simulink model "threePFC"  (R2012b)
settings: Solver=ode15s  StartTime=0.0  StopTime=0.1  MaxStep=1e-6  RelTol=1e-4
libraries: powerlib x29, simulink x10

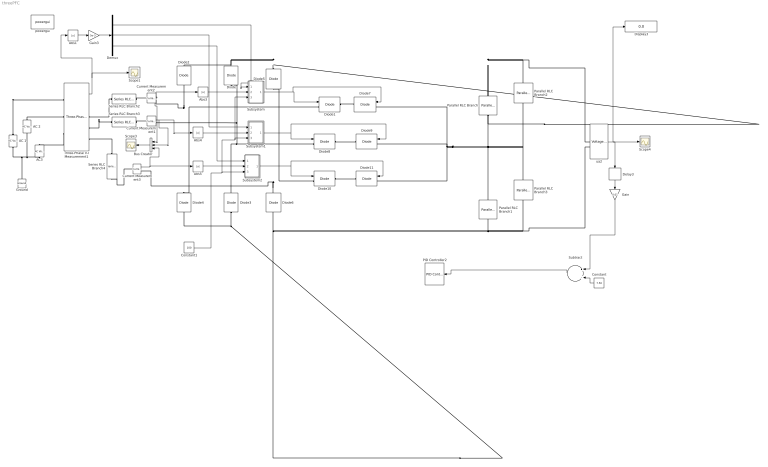
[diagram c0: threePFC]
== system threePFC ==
  AC 1 : powerlib/Electrical Sources/AC Voltage Source  Amplitude=200  Phase=0  Frequency=50  SampleTime=0  Measurements=Voltage
  AC 2 : powerlib/Electrical Sources/AC Voltage Source  Amplitude=200  Phase=120  Frequency=50  SampleTime=0  Measurements=None
  AC3 : powerlib/Electrical Sources/AC Voltage Source  Amplitude=200  Phase=240  Frequency=50  SampleTime=0  Measurements=None
  Abs{1,3..5} (4 alike) : Abs
  Bus Creator : BusCreator  Inputs=3
  Constant : Constant  Value=7.50
  Constant1 : Constant  Value=100
  Current Measurement1 : powerlib/Measurements/Current Measurement  PhasorSimulation=off  OutputType=Complex  PSBequivalent=0
  Current Measurement2 : powerlib/Measurements/Current Measurement  PhasorSimulation=off  OutputType=Complex  PSBequivalent=0
  Current Measurement3 : powerlib/Measurements/Current Measurement  PhasorSimulation=off  OutputType=Complex  PSBequivalent=0
  Delay3 : Delay  DelayLength=1  InitialCondition=0  SampleTime=1e-6
  Demux : Demux  Outputs=3
  Diode{,2..6} (6 alike) : powerlib/Power Electronics/Diode  Ron=0.001  Lon=0  Vf=0.8  IC=0  UseSnubber=off  Rs=500  Cs=250e-9  Measurements=off
  Diode{1,7..11} (6 alike) : powerlib/Power Electronics/IGBT//Diode  Ron=1e-3  Rs=1e5  Cs=inf  Measurements=off
  Display3 : Display
  Gain : Gain  Gain=0.01
  Gain3 : Gain  Gain=5e-3
  Ground : powerlib/Elements/Ground  LConnTagsString=a
  PID Controller2 : simulink/Continuous/PID Controller  Controller=PID  TimeDomain=Continuous-time  SampleTime=1  IntegratorMethod=Forward Euler  FilterMethod=Forward Euler  Form=Parallel  P=2.0  I=1.0  D=0  N=100  InitialConditionSource=internal  InitialConditionForIntegrator=0  InitialConditionForFilter=0  ExternalReset=none  ZeroCross=off  LimitOutput=on  UpperSaturationLimit=inf  LowerSaturationLimit=-inf  LinearizeAsGain=on  AntiWindupMode=back-calculation  Kb=10  TrackingMode=off  Kt=1  PParamMin=[]  PParamMax=[]  IParamMin=[]  IParamMax=[]  DParamMin=[]  DParamMax=[]  NParamMin=[]  NParamMax=[]  KbParamMin=[]  KbParamMax=[]  KtParamMin=[]  KtParamMax=[]  POutMin=[]  POutMax=[]  IOutMin=[]  IOutMax=[]  DOutMin=[]  DOutMax=[]  NOutMin=[]  NOutMax=[]  KbOutMin=[]  KbOutMax=[]  KtOutMin=[]  KtOutMax=[]  IntegratorOutMin=[]  IntegratorOutMax=[]  FilterOutMin=[]  FilterOutMax=[]  SumOutMin=[]  SumOutMax=[]  SumI1OutMin=[]  SumI1OutMax=[]  SumI2OutMin=[]  SumI2OutMax=[]  SumI3OutMin=[]  SumI3OutMax=[]  SumDOutMin=[]  SumDOutMax=[]  SaturationOutMin=[]  SaturationOutMax=[]  IntegratorContinuousStateAttributes=''  IntegratorStateMustResolveToSignalObject=off  IntegratorRTWStateStorageClass=Auto  FilterContinuousStateAttributes=''  FilterStateMustResolveToSignalObject=off  FilterRTWStateStorageClass=Auto
  Parallel RLC Branch : powerlib/Elements/Parallel RLC Branch  LConnTagsString=a  RConnTagsString=__new0  BranchType=C  Resistance=50  Inductance=1e-3  SetiL0=off  InitialCurrent=0  Capacitance=3000e-6  Setx0=on  InitialVoltage=200  Measurements=None
  Parallel RLC Branch1 : powerlib/Elements/Parallel RLC Branch  LConnTagsString=a  RConnTagsString=__new0  BranchType=C  Resistance=50  Inductance=1e-3  SetiL0=off  InitialCurrent=0  Capacitance=3000e-6  Setx0=on  InitialVoltage=200  Measurements=None
  Parallel RLC Branch2 : powerlib/Elements/Parallel RLC Branch  LConnTagsString=a  RConnTagsString=__new0  BranchType=R  Resistance=80  Inductance=1e-3  SetiL0=off  InitialCurrent=0  Capacitance=500e-6  Setx0=off  InitialVoltage=0  Measurements=None
  Parallel RLC Branch3 : powerlib/Elements/Parallel RLC Branch  LConnTagsString=a  RConnTagsString=__new0  BranchType=R  Resistance=80  Inductance=1e-3  SetiL0=off  InitialCurrent=0  Capacitance=500e-6  Setx0=off  InitialVoltage=0  Measurements=None
  Scope1 : Scope
  Scope3 : Scope
  Scope4 : Scope
  Series RLC Branch2 : powerlib/Elements/Series RLC Branch  LConnTagsString=__new0  RConnTagsString=__new0  BranchType=L  Resistance=1  Inductance=150e-6  SetiL0=off  InitialCurrent=0  Capacitance=1e-6  Setx0=off  InitialVoltage=0  Measurements=None
  Series RLC Branch3 : powerlib/Elements/Series RLC Branch  LConnTagsString=__new0  RConnTagsString=__new0  BranchType=L  Resistance=1  Inductance=150e-6  SetiL0=off  InitialCurrent=0  Capacitance=1e-6  Setx0=off  InitialVoltage=0  Measurements=None
  Series RLC Branch4 : powerlib/Elements/Series RLC Branch  LConnTagsString=__new0  RConnTagsString=__new0  BranchType=L  Resistance=1  Inductance=150e-6  SetiL0=off  InitialCurrent=0  Capacitance=1e-6  Setx0=off  InitialVoltage=0  Measurements=None
  Subsystem : Subsystem
  Subsystem1 : Subsystem
  Subsystem2 : Subsystem
  Subtract : Sum  Inputs=-+
  Three-Phase V-I Measurement1 : powerlib/Measurements/Three-Phase V-I Measurement  VoltageMeasurement=phase-to-ground  SetLabelV=off  LabelV=Vabc  Vpu=off  VpuLL=off  CurrentMeasurement=yes  SetLabelI=off  LabelI=Iabc  Ipu=off  Pbase=100e6  Vbase=500e3  OutputType=Complex  PhasorSimulation=off  PSBequivalent=0
  powergui : powerlib/powergui  Priority=1  SimulationMode=Continuous  SolverType=Tustin  SampleTime=5e-6  frequency=60  SPID=off  DisableSnubberDevices=off  DisableRonSwitches=off  DisableVfSwitches=off  SwTol=0  Interpol=off  DisplayEquations=off  FunctionMessages=off  frequencyindice=50  Pbase=100e6  ErrMax=1e-4  Iterations=50  UnitsV=kV  UnitsW=MW  echomessages=off  HookPort=off  EnableUseOfTLC=off  x0status=blocks  RestoreLinks=warning  ResistiveCurrentMeasurement=off  Ylog=off  Xlog=on  ShowGrid=off  save=off  variable=ZData  ZoomFFT=off  StartTime=0.0  cycles=1  DisplayStyle=1  FreqAxis=off  MaxFrequency=1000  frequencyindicesteady=1  display=off  methode=off
  ua2 : powerlib/Measurements/Voltage Measurement  PhasorSimulation=off  OutputType=Complex  PSBequivalent=0
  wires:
  Constant/1 -> Subtract/2
  ua2/1 -> Delay3/1, Scope4/1, Display3/1
  Gain/1 -> Subtract/1
  Subtract/1 -> PID Controller2/1
  Delay3/1 -> Gain/1
  Current Measurement2/1 -> Abs3/1, Bus Creator/1
  Abs3/1 -> Subsystem/2(Iin)
  Abs4/1 -> Subsystem1/2(Iin)
  Demux/2 -> Subsystem1/1(Vac)
  Demux/3 -> Subsystem2/1(Vac)
  Demux/1 -> Subsystem/1(Vac)
  Current Measurement1/1 -> Abs4/1, Bus Creator/2
  Abs5/1 -> Subsystem2/2(Iin)
  Current Measurement3/1 -> Bus Creator/3, Abs5/1
  Gain3/1 -> Demux/1
  Abs1/1 -> Gain3/1
  Three-Phase V-I Measurement1/1 -> Scope1/1, Abs1/1
  Subsystem/1(Out1) -> Diode7/1, Diode1/1
  Subsystem1/1(Out1) -> Diode8/1, Diode9/1
  Subsystem2/1(Out1) -> Diode10/1, Diode11/1
  Bus Creator/1 -> Scope3/1
  Constant1/1 -> Subsystem/3(Iref), Subsystem1/3(Iref), Subsystem2/3("Iref ")
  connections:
  AC 1/LConn1 -- AC3/LConn1 -- AC 2/LConn1 -- Ground/LConn1
  AC 1/RConn1 -- Three-Phase V-I Measurement1/LConn1
  AC 2/RConn1 -- Three-Phase V-I Measurement1/LConn2
  Diode8/LConn1 -- Diode3/RConn1 -- Diode/LConn1 -- Current Measurement1/RConn1
  Diode10/LConn1 -- Current Measurement3/RConn1 -- Diode6/RConn1 -- Diode5/LConn1
  Diode5/RConn1 -- Parallel RLC Branch2/LConn1 -- ua2/LConn1 -- Parallel RLC Branch/LConn1 -- Diode2/RConn1 -- Diode/RConn1
  Diode3/LConn1 -- ua2/LConn2 -- Parallel RLC Branch3/RConn1 -- Parallel RLC Branch1/RConn1 -- Diode6/LConn1 -- Diode4/LConn1
  Diode1/LConn1 -- Diode2/LConn1 -- Current Measurement2/RConn1 -- Diode4/RConn1
  Diode1/RConn1 -- Diode7/RConn1
  Diode8/RConn1 -- Diode9/RConn1
  Diode10/RConn1 -- Diode11/RConn1
  Three-Phase V-I Measurement1/LConn3 -- AC3/RConn1
  Series RLC Branch2/LConn1 -- Three-Phase V-I Measurement1/RConn1
  Three-Phase V-I Measurement1/RConn2 -- Series RLC Branch3/LConn1
  Series RLC Branch4/LConn1 -- Three-Phase V-I Measurement1/RConn3
  Diode11/LConn1 -- Diode9/LConn1 -- Diode7/LConn1 -- Parallel RLC Branch3/LConn1 -- Parallel RLC Branch2/RConn1 -- Parallel RLC Branch/RConn1 -- Parallel RLC Branch1/LConn1
  Series RLC Branch2/RConn1 -- Current Measurement2/LConn1
  Series RLC Branch3/RConn1 -- Current Measurement1/LConn1
  Current Measurement3/LConn1 -- Series RLC Branch4/RConn1

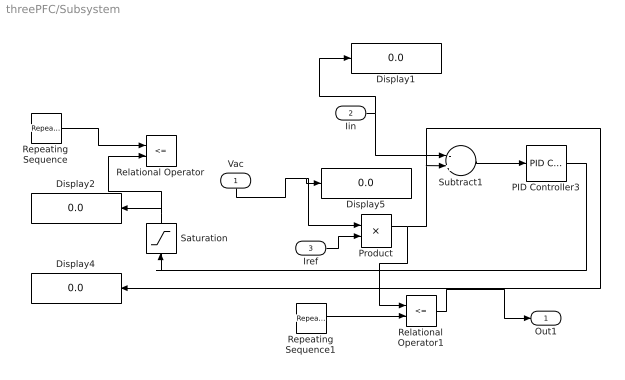
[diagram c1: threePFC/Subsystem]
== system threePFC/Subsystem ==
  Vac : Inport
  Iin : Inport  Port=2
  Iref : Inport  Port=3
  Display{1..2,4..5} (4 alike) : Display
  PID Controller3 : simulink/Continuous/PID Controller  Controller=PID  TimeDomain=Continuous-time  SampleTime=1  IntegratorMethod=Forward Euler  FilterMethod=Forward Euler  Form=Parallel  P=1  I=0  D=0  N=100  InitialConditionSource=internal  InitialConditionForIntegrator=0  InitialConditionForFilter=0  ExternalReset=none  ZeroCross=off  LimitOutput=on  UpperSaturationLimit=inf  LowerSaturationLimit=-inf  LinearizeAsGain=on  AntiWindupMode=back-calculation  Kb=10  TrackingMode=off  Kt=1  PParamMin=[]  PParamMax=[]  IParamMin=[]  IParamMax=[]  DParamMin=[]  DParamMax=[]  NParamMin=[]  NParamMax=[]  KbParamMin=[]  KbParamMax=[]  KtParamMin=[]  KtParamMax=[]  POutMin=[]  POutMax=[]  IOutMin=[]  IOutMax=[]  DOutMin=[]  DOutMax=[]  NOutMin=[]  NOutMax=[]  KbOutMin=[]  KbOutMax=[]  KtOutMin=[]  KtOutMax=[]  IntegratorOutMin=[]  IntegratorOutMax=[]  FilterOutMin=[]  FilterOutMax=[]  SumOutMin=[]  SumOutMax=[]  SumI1OutMin=[]  SumI1OutMax=[]  SumI2OutMin=[]  SumI2OutMax=[]  SumI3OutMin=[]  SumI3OutMax=[]  SumDOutMin=[]  SumDOutMax=[]  SaturationOutMin=[]  SaturationOutMax=[]  IntegratorContinuousStateAttributes=''  IntegratorStateMustResolveToSignalObject=off  IntegratorRTWStateStorageClass=Auto  FilterContinuousStateAttributes=''  FilterStateMustResolveToSignalObject=off  FilterRTWStateStorageClass=Auto
  Product : Product
  Relational Operator : RelationalOperator  Operator=<=  OutDataTypeStr=boolean
  Relational Operator1 : RelationalOperator  Operator=<=  OutDataTypeStr=boolean
  Repeating Sequence : simulink/Sources/Repeating Sequence  rep_seq_t=[0 5e-6]  rep_seq_y=[0 20]
  Repeating Sequence1 : simulink/Sources/Repeating Sequence  rep_seq_t=[0 1e-5]  rep_seq_y=[0 100]
  Saturation : Saturate  UpperLimit=inf  LowerLimit=-inf
  Subtract1 : Sum  Inputs=-+
  Out1 : Outport
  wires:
  Vac/1 -> Product/1, Display5/1
  Saturation/1 -> Relational Operator/2, Display2/1
  Subtract1/1 -> PID Controller3/1
  Product/1 -> Relational Operator1/1, Subtract1/2, Display4/1
  Repeating Sequence/1 -> Relational Operator/1
  PID Controller3/1 -> Saturation/1
  Iin/1 -> Subtract1/1, Display1/1
  Iref/1 -> Product/2
  Repeating Sequence1/1 -> Relational Operator1/2
  Relational Operator1/1 -> Out1/1

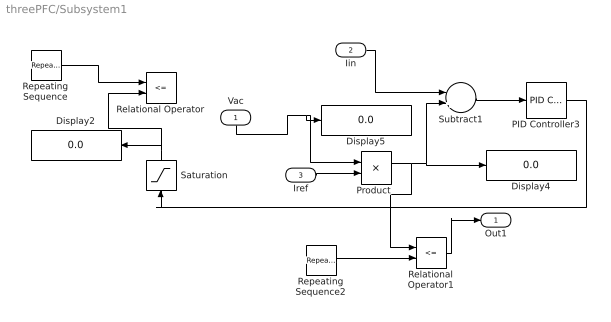
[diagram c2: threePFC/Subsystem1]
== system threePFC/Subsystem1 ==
  Vac : Inport
  Iin : Inport  Port=2
  Iref : Inport  Port=3
  Display2 : Display
  Display4 : Display
  Display5 : Display
  PID Controller3 : simulink/Continuous/PID Controller  Controller=PID  TimeDomain=Continuous-time  SampleTime=1  IntegratorMethod=Forward Euler  FilterMethod=Forward Euler  Form=Parallel  P=1  I=0  D=0  N=100  InitialConditionSource=internal  InitialConditionForIntegrator=0  InitialConditionForFilter=0  ExternalReset=none  ZeroCross=off  LimitOutput=on  UpperSaturationLimit=inf  LowerSaturationLimit=-inf  LinearizeAsGain=on  AntiWindupMode=back-calculation  Kb=10  TrackingMode=off  Kt=1  PParamMin=[]  PParamMax=[]  IParamMin=[]  IParamMax=[]  DParamMin=[]  DParamMax=[]  NParamMin=[]  NParamMax=[]  KbParamMin=[]  KbParamMax=[]  KtParamMin=[]  KtParamMax=[]  POutMin=[]  POutMax=[]  IOutMin=[]  IOutMax=[]  DOutMin=[]  DOutMax=[]  NOutMin=[]  NOutMax=[]  KbOutMin=[]  KbOutMax=[]  KtOutMin=[]  KtOutMax=[]  IntegratorOutMin=[]  IntegratorOutMax=[]  FilterOutMin=[]  FilterOutMax=[]  SumOutMin=[]  SumOutMax=[]  SumI1OutMin=[]  SumI1OutMax=[]  SumI2OutMin=[]  SumI2OutMax=[]  SumI3OutMin=[]  SumI3OutMax=[]  SumDOutMin=[]  SumDOutMax=[]  SaturationOutMin=[]  SaturationOutMax=[]  IntegratorContinuousStateAttributes=''  IntegratorStateMustResolveToSignalObject=off  IntegratorRTWStateStorageClass=Auto  FilterContinuousStateAttributes=''  FilterStateMustResolveToSignalObject=off  FilterRTWStateStorageClass=Auto
  Product : Product
  Relational Operator : RelationalOperator  Operator=<=  OutDataTypeStr=boolean
  Relational Operator1 : RelationalOperator  Operator=<=  OutDataTypeStr=boolean
  Repeating Sequence : simulink/Sources/Repeating Sequence  rep_seq_t=[0 5e-6]  rep_seq_y=[0 50]
  Repeating Sequence2 : simulink/Sources/Repeating Sequence  rep_seq_t=[0 1e-5]  rep_seq_y=[0 100]
  Saturation : Saturate  UpperLimit=inf  LowerLimit=0
  Subtract1 : Sum  Inputs=-+
  Out1 : Outport
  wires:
  Vac/1 -> Product/1, Display5/1
  Saturation/1 -> Relational Operator/2, Display2/1
  Subtract1/1 -> PID Controller3/1
  Product/1 -> Relational Operator1/1, Subtract1/2, Display4/1
  Repeating Sequence/1 -> Relational Operator/1
  PID Controller3/1 -> Saturation/1
  Iin/1 -> Subtract1/1
  Iref/1 -> Product/2
  Repeating Sequence2/1 -> Relational Operator1/2
  Relational Operator1/1 -> Out1/1

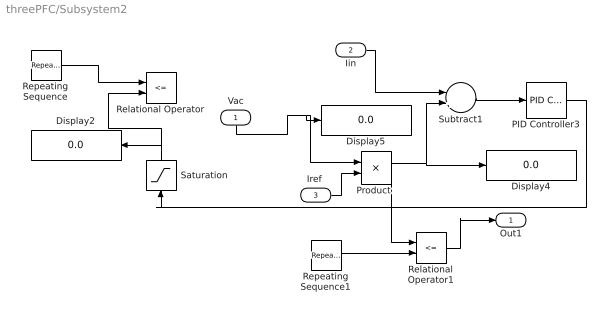
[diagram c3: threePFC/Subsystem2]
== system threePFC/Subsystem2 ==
  Vac : Inport
  Iin : Inport  Port=2
  "Iref " : Inport  Port=3
  Display2 : Display
  Display4 : Display
  Display5 : Display
  PID Controller3 : simulink/Continuous/PID Controller  Controller=PID  TimeDomain=Continuous-time  SampleTime=1  IntegratorMethod=Forward Euler  FilterMethod=Forward Euler  Form=Parallel  P=1  I=0  D=0  N=100  InitialConditionSource=internal  InitialConditionForIntegrator=0  InitialConditionForFilter=0  ExternalReset=none  ZeroCross=off  LimitOutput=on  UpperSaturationLimit=inf  LowerSaturationLimit=-inf  LinearizeAsGain=on  AntiWindupMode=back-calculation  Kb=10  TrackingMode=off  Kt=1  PParamMin=[]  PParamMax=[]  IParamMin=[]  IParamMax=[]  DParamMin=[]  DParamMax=[]  NParamMin=[]  NParamMax=[]  KbParamMin=[]  KbParamMax=[]  KtParamMin=[]  KtParamMax=[]  POutMin=[]  POutMax=[]  IOutMin=[]  IOutMax=[]  DOutMin=[]  DOutMax=[]  NOutMin=[]  NOutMax=[]  KbOutMin=[]  KbOutMax=[]  KtOutMin=[]  KtOutMax=[]  IntegratorOutMin=[]  IntegratorOutMax=[]  FilterOutMin=[]  FilterOutMax=[]  SumOutMin=[]  SumOutMax=[]  SumI1OutMin=[]  SumI1OutMax=[]  SumI2OutMin=[]  SumI2OutMax=[]  SumI3OutMin=[]  SumI3OutMax=[]  SumDOutMin=[]  SumDOutMax=[]  SaturationOutMin=[]  SaturationOutMax=[]  IntegratorContinuousStateAttributes=''  IntegratorStateMustResolveToSignalObject=off  IntegratorRTWStateStorageClass=Auto  FilterContinuousStateAttributes=''  FilterStateMustResolveToSignalObject=off  FilterRTWStateStorageClass=Auto
  Product : Product
  Relational Operator : RelationalOperator  Operator=<=  OutDataTypeStr=boolean
  Relational Operator1 : RelationalOperator  Operator=<=  OutDataTypeStr=boolean
  Repeating Sequence : simulink/Sources/Repeating Sequence  rep_seq_t=[0 5e-6]  rep_seq_y=[0 50]
  Repeating Sequence1 : simulink/Sources/Repeating Sequence  rep_seq_t=[0 1e-5]  rep_seq_y=[0 100]
  Saturation : Saturate  UpperLimit=inf  LowerLimit=0
  Subtract1 : Sum  Inputs=-+
  Out1 : Outport
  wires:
  Vac/1 -> Product/1, Display5/1
  Saturation/1 -> Relational Operator/2, Display2/1
  Subtract1/1 -> PID Controller3/1
  Product/1 -> Subtract1/2, Display4/1, Relational Operator1/1
  Repeating Sequence/1 -> Relational Operator/1
  PID Controller3/1 -> Saturation/1
  Iin/1 -> Subtract1/1
  "Iref "/1 -> Product/2
  Repeating Sequence1/1 -> Relational Operator1/2
  Relational Operator1/1 -> Out1/1
